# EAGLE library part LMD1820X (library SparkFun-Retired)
LMD1820X H-Bridge - BOB-00747
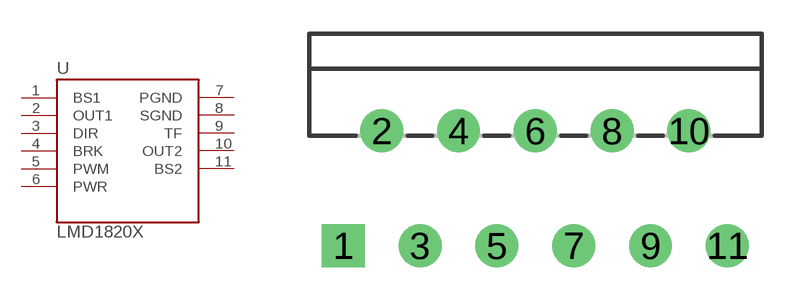
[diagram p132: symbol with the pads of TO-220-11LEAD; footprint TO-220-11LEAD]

Designator prefix -

## LMD1820X  [TO-220-11LEAD]
1  BS1
2  OUT1
3  DIR
4  BRK
5  PWM
6  PWR
7  PGND
8  SGND
9  TF
10  OUT2
11  BS2

## Footprint TO-220-11LEAD (pad centres in mm)
TO-220 11 Pin Package
drill 1.1 pad 1.9 square: 1 1.5,-4.87
drill 1.1 pad 1.9: 2 3.2,0.21; 3 4.9,-4.87; 4 6.6,0.21; 5 8.3,-4.87; 6 10,0.21; 7 11.7,-4.87; 8 13.4,0.21; 9 15.1,-4.87; 10 16.8,0.21; 11 18.5,-4.87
